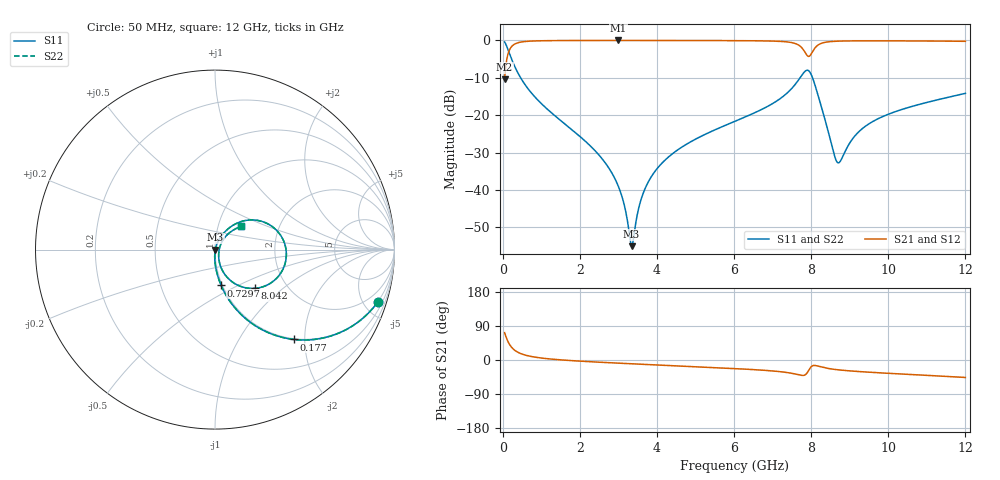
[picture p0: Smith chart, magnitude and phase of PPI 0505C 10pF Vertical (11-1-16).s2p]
# GHz S MA R 50
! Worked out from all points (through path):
!   1601 points, 50 MHz to 12 GHz, reference 50 ohm
!   highest |S21| = -0.02 dB at 3 GHz (marker M1); lowest = -10.4 dB at 50 MHz (marker M2)
!   group delay of S21, straight-line fit = 13.2 ps
!   lowest |S11| = -55.0 dB at 3.344 GHz (marker M3), VSWR 1.00, Z = 50.2 - j0.0425 ohm
!   |S11| at or under -10 dB: 465.5 MHz to 7.712 GHz (7.246 GHz wide, 177 % of centre); 8.036 GHz to end of sweep
!   |S22| runs from -55.0 to -0.4 dB; largest |S21 - S12| = 0
!   S11 on the Smith chart (normalised r, x): 50 MHz: 0.98, -6.27; 177 MHz: 0.98, -1.77; 729.7 MHz: 0.99, -0.41; 8.042 GHz: 1.39, -0.66; 12 GHz: 1.29, +0.35
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0.05  0.9534 -17.7  0.3016 72.3  0.3016 72.3  0.9534 -17.7
0.1769688  0.6651 -48.8  0.7464 41.2  0.7464 41.2  0.6651 -48.8
0.3636875  0.3948 -67.8  0.9182 22.2  0.9182 22.2  0.3948 -67.8
0.7296563  0.2027 -80.3  0.9784 9.5  0.9784 9.5  0.2027 -80.3
2.044156  0.04986 -91.7  0.9973 -3.3  0.9973 -3.3  0.04986 -91.7
2.634187  0.02404 -92.8  0.998 -6.5  0.998 -6.5  0.02404 -92.8
3.000156  0.01118 -89.8  0.9981 -8.3  0.9981 -8.3  0.01118 -89.8
3.343719  0.001775 -13.8  0.998 -10.0  0.998 -10.0  0.001775 -13.8
3.635  0.008785 66.4  0.9979 -11.3  0.9979 -11.3  0.008785 66.4
4.038312  0.02026 71.1  0.9975 -13.2  0.9975 -13.2  0.02026 71.1
4.762781  0.0408 70.2  0.9965 -16.5  0.9965 -16.5  0.0408 70.2
6.025  0.08298 64.8  0.9925 -22.6  0.9925 -22.6  0.08298 64.8
7.093031  0.1531 55.6  0.9754 -29.7  0.9754 -29.7  0.1531 55.6
7.660656  0.29 34.0  0.8739 -38.7  0.8739 -38.7  0.29 34.0
7.87725  0.3972 -1.6  0.6471 -36.3  0.6471 -36.3  0.3972 -1.6
8.019156  0.3331 -39.0  0.684 -16.2  0.684 -16.2  0.3331 -39.0
8.041562  0.3108 -44.0  0.7161 -15.0  0.7161 -15.0  0.3108 -44.0
8.250687  0.1375 -69.4  0.9077 -18.1  0.9077 -18.1  0.1375 -69.4
8.691344  0.02313 -14.4  0.9768 -25.8  0.9768 -25.8  0.02313 -14.4
9.2515  0.06118 49.1  0.9866 -30.6  0.9866 -30.6  0.06118 49.1
10.01331  0.1036 50.7  0.9866 -35.2  0.9866 -35.2  0.1036 50.7
12  0.196 41.6  0.9719 -46.1  0.9719 -46.1  0.196 41.6
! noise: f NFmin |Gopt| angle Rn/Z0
0.05  0.0003987  0.8734  1.895  0.0006791
1.372  0.003999  0.6751  4.544  0.00237
2.701  0.006638  0.6264  8.212  0.003311
4.031  0.009187  0.604  11.87  0.004241
5.36  0.01241  0.6103  15.5  0.005802
6.682  0.02096  0.6983  19.33  0.01321
8.012  0.1911  0.9546  23.61  0.9077
9.341  0.03085  0.7145  27.16  0.02019
10.67  0.02682  0.6434  30.34  0.0133
12  0.03106  0.6547  33.72  0.01576
